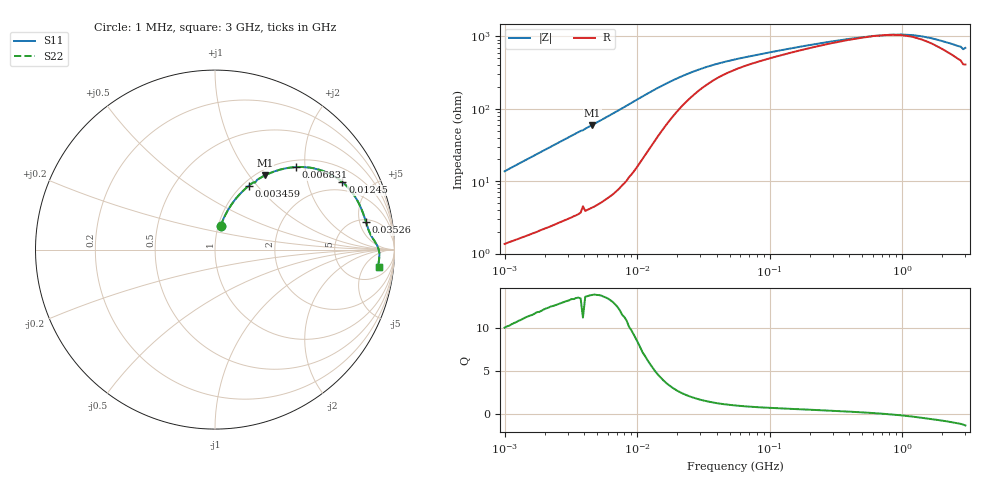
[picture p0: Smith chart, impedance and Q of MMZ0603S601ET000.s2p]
! S-Parameter Data Generated by TDK Corporation
! Copyright(C) 2025 TDK Corporation.
! All Rights Reserved.
! TDK P/N: MMZ0603S601ET000 (Chip Bead)
! Property: |Z|=600ohm at 100MHz
! Size(LxWxT): 0.6x0.3x0.3mm
! Model Type: s2p (Touchstone File Format Version 1.0)
! Frequency: DC=Yes Start=1MHz Stop=3000MHz 202points Log-sweep
! Model Generated on Feb. 6, 2025
! Terms and conditions regarding TDK Simulation Models:
! 1)This simulation model is being provided solely for informational
!  purposes. Please refer to the specifications of the products in
!  terms of detailed characteristics of such products.
! 2)In no event shall TDK Corporation of any of its subsidiaries be
!  liable for any loss or damage arising, directly or indirectly,
!  from any information contained in this simulation model, including,
!  but not limited to loss or damages arising from any inaccuracies,
!  omissions or errors in connection with such information.
! 3)Any and all copyrights on this simulation model are owned by
!  TDK Corporation.  Duplication or redistribution of this simulation
!  model without prior written permission from TDK Corporation
!  is prohibited.
! 4)This simulation model is subject to any modification or change
!  without any prior notice.
! 5)Neither TDK Corporation nor any of its subsidiaries shall make any
!  warranty, express or implied, including but not limited to the
!  correctness, implied warranties of merchantability and fitness for
!  a particular purpose with respect to this simulation models.
! 6)The use of this simulation model shall be deemed to have consented
!  to the terms and conditions hereof.
! Port Assignments:
!  1 ---@@@--- 2
! Applicable Conditions:
!  Temperature = 25 degC
!  DC Bias Current = 0 A
!  Small Signal Operation
# Hz S MA R 50
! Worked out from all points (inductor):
!   201 points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, 1 MHz to 3 GHz, reference 50 ohm
!   read as one part in series: L = 2.16 uH near 1.041 MHz
!   highest Q = 13.8 at 4.578 MHz (marker M1), where L = 2.07 uH
!   self-resonance near 701.1 MHz
!   S11 on the Smith chart (normalised r, x): 1 MHz: 1.03, +0.27; 3.459 MHz: 1.07, +0.91; 6.831 MHz: 1.14, +1.79; 12.45 MHz: 1.57, +3.33; 35.26 MHz: 5.58, +6.32; 3 GHz: 9, -11
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1000000  0.1338 76.7  0.9778 -7.7  0.9778 -7.7  0.1338 76.7
1974946  0.2515 70.8  0.9475 -14.5  0.9475 -14.5  0.2515 70.8
2613693  0.3207 66.9  0.9226 -18.6  0.9226 -18.6  0.3207 66.9
3459026  0.4039 62.0  0.8854 -23.8  0.8854 -23.8  0.4039 62.0
3900413  0.436 59.2  0.862 -25.7  0.862 -25.7  0.436 59.2
4577760  0.4977 56.1  0.8323 -29.8  0.8323 -29.8  0.4977 56.1
6831390  0.643 45.7  0.7173 -39.9  0.7173 -39.9  0.643 45.7
9040831  0.7332 37.3  0.6092 -46.8  0.6092 -46.8  0.7332 37.3
1.245355e7  0.8033 27.9  0.4753 -52.4  0.4753 -52.4  0.8033 27.9
1.461624e7  0.8228 23.9  0.4149 -53.4  0.4149 -53.4  0.8228 23.9
2.095589e7  0.8442 16.7  0.3087 -51.7  0.3087 -51.7  0.8442 16.7
3.526298e7  0.8556 10.2  0.2191 -43.9  0.2191 -43.9  0.8556 10.2
5.477226e7  0.8629 7.1  0.1792 -36.6  0.1792 -36.6  0.8629 7.1
2.136344e8  0.8936 2.7  0.1151 -21.2  0.1151 -21.2  0.8936 2.7
4.570858e8  0.9067 1.0  0.09481 -9.7  0.09481 -9.7  0.9067 1.0
8.005644e8  0.9135 -0.3  0.08667 3.6  0.08667 3.6  0.9135 -0.3
1.059487e9  0.916 -1.2  0.08645 13.0  0.08645 13.0  0.916 -1.2
1.402151e9  0.9167 -2.2  0.09123 23.0  0.09123 23.0  0.9167 -2.2
2.266846e9  0.9149 -4.5  0.1131 39.0  0.1131 39.0  0.9149 -4.5
2.769173e9  0.9139 -5.6  0.1265 44.4  0.1265 44.4  0.9139 -5.6
2.882277e9  0.9097 -6.2  0.1365 45.6  0.1365 45.6  0.9097 -6.2
3e9  0.9167 -6.1  0.1319 47.8  0.1319 47.8  0.9167 -6.1
